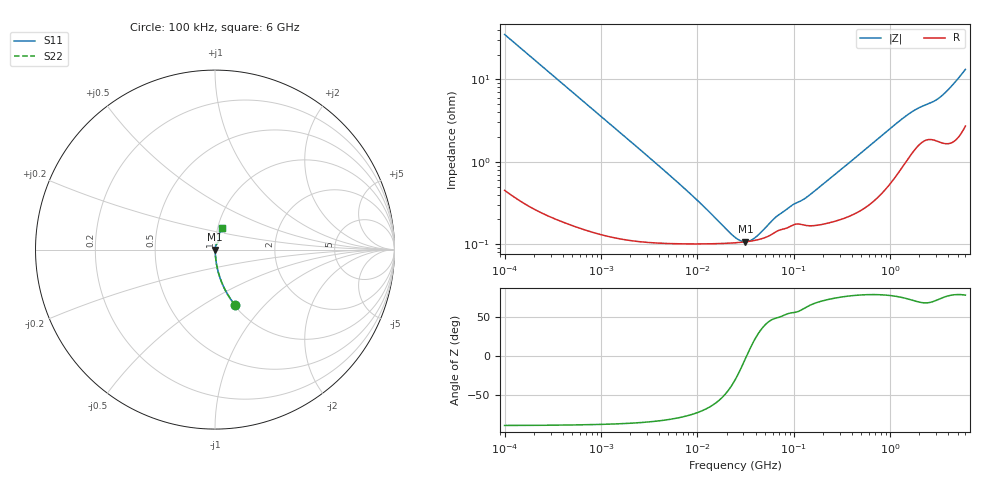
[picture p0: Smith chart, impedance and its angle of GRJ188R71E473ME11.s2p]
!Murata Part Number: GRJ188R71E473ME11
!These Parameters are Measured in Series Mode Connection
!Data Generated on Jun 19, 2026
!  o--ll--o
!Port1  Port2
!  o------o
!Operation Temp=25[degC], DC Bias Voltage=0[V]
!Freq. Start=100[kHz] Stop=6[GHz] 401[Steps]
# Hz S RI R 50
!Freq.(Hz) S11(Real) S11(Imag) S21(Real) S21(Imag) S12(Real) S12(Imag) S22(Real) S22(Imag)
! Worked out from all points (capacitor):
!   401 points, 100 kHz to 6 GHz, reference 50 ohm
!   read as one part in series: C = 45.3 nF near 105.7 kHz
!   lowest |Z| = 107 mohm at 31.38 MHz (marker M1)
!   series resonance near 32.33 MHz, so ESL is about 530 pH
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100000  0.1126 -0.3098  0.8874 0.3098  0.8874 0.3098  0.1126 -0.3098
151071  0.0541 -0.2194  0.9459 0.2194  0.9459 0.2194  0.0541 -0.2194
241130  0.0232 -0.1424  0.9768 0.1424  0.9768 0.1424  0.0232 -0.1424
374436  0.0107 -0.0932  0.9893 0.0932  0.9893 0.0932  0.0107 -0.0932
631452  0.00466 -0.0558  0.9953 0.0558  0.9953 0.0558  0.00466 -0.0558
1402027  0.00183 -0.0253  0.9982 0.0253  0.9982 0.0253  0.00183 -0.0253
3987316  0.00111 -0.00882  0.9989 0.00882  0.9989 0.00882  0.00111 -0.00882
9353785  0.00102 -0.0035  0.999 0.0035  0.999 0.0035  0.00102 -0.0035
2.517799e7  0.00104 -0.000558  0.999 0.000558  0.999 0.000558  0.00104 -0.000558
2.810622e7  0.00105 -0.00031  0.9989 0.00031  0.9989 0.00031  0.00105 -0.00031
3.137502e7  0.00107 -6.62e-05  0.9989 6.62e-05  0.9989 6.62e-05  0.00107 -6.62e-05
3.502398e7  0.00108 0.000177  0.9989 -0.000177  0.9989 -0.000177  0.00108 0.000177
3.909733e7  0.00111 0.000422  0.9989 -0.000422  0.9989 -0.000422  0.00111 0.000422
6.777267e7  0.00145 0.00168  0.9985 -0.00168  0.9985 -0.00168  0.00145 0.00168
9.427557e7  0.00167 0.00241  0.9983 -0.00241  0.9983 -0.00241  0.00167 0.00241
1.241232e8  0.00172 0.003  0.9983 -0.003  0.9983 -0.003  0.00172 0.003
1.546735e8  0.00168 0.00382  0.9983 -0.00382  0.9983 -0.00382  0.00168 0.00382
9.76689e8  0.00581 0.024  0.9942 -0.024  0.9942 -0.024  0.00581 0.024
1.693027e9  0.0141 0.0376  0.9859 -0.0376  0.9859 -0.0376  0.0141 0.0376
3.187187e9  0.0202 0.0546  0.9798 -0.0546  0.9798 -0.0546  0.0202 0.0546
3.971646e9  0.0213 0.0702  0.9787 -0.0702  0.9787 -0.0702  0.0213 0.0702
6e9  0.0416 0.1207  0.9584 -0.1207  0.9584 -0.1207  0.0416 0.1207
